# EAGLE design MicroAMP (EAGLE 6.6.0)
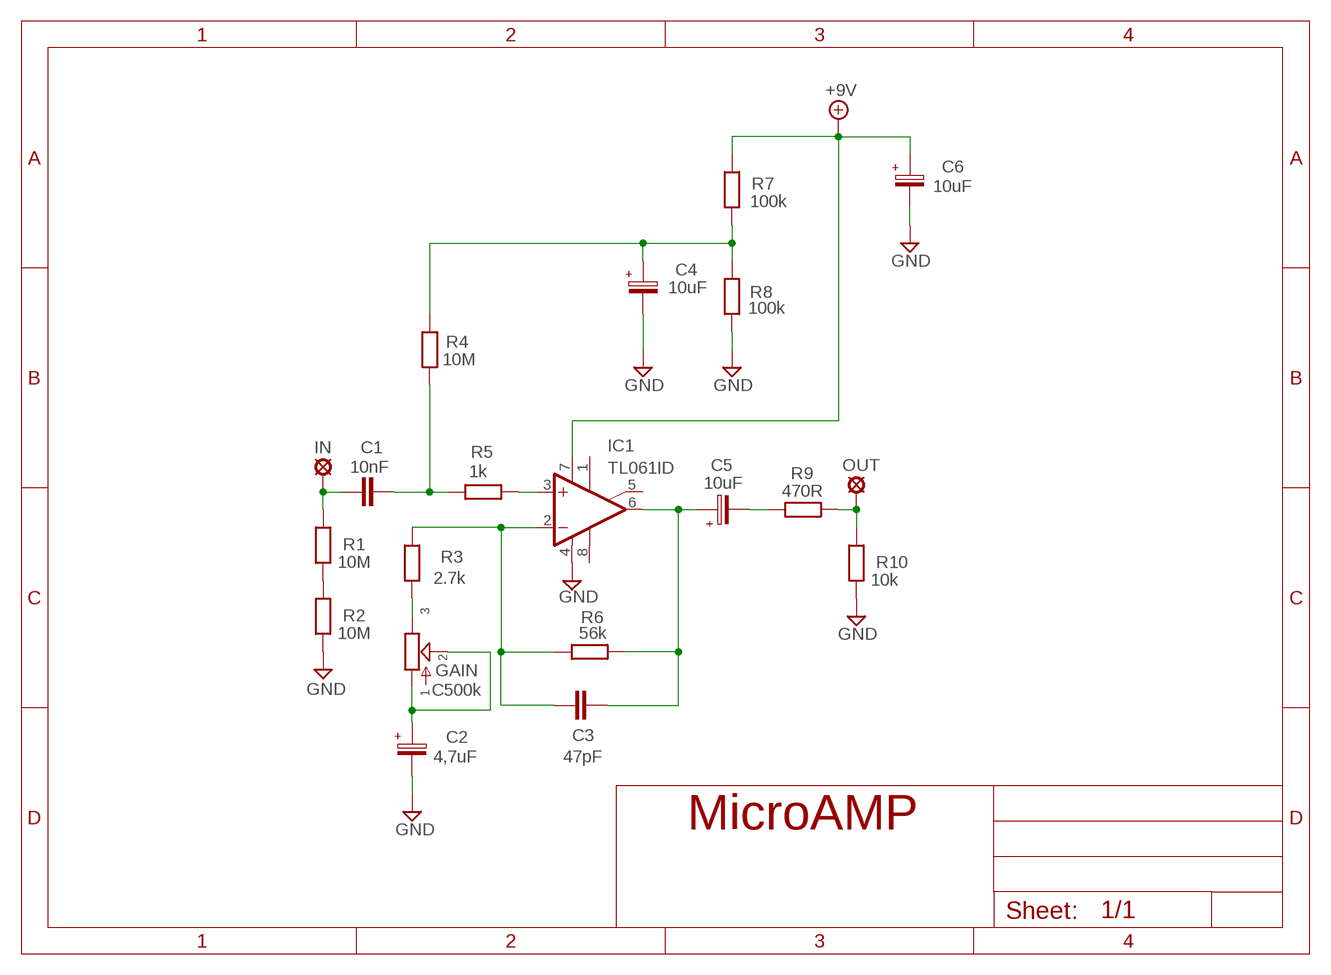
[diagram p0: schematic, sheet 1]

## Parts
+9V  +9V  +9V(T)1  [ROUND]
C1  10nF  1NF-15NF  [3,5MM]
C2  4,7uF  063-EU  [063_025]
C3  47pF  050X030_0501  [050X030_050_1]
C4  10uF  063-EU  [063_025]
C5  10uF  063-EU  [063_025]
C6  10uF  063-EU  [063_025]
GAIN  C500k  POT-EU16MM  [16MM]
GND  GND  GND(T)1  [ROUND]
GND7  GND  GND(T)1  [ROUND]
IC1  TL061ID  TL071D  [SO08]
IN  MCS10B  [MCS10B]
OUT  MCS10B  [MCS10B]
R1  10M  6MM-EU3  [R0207/3]
R2  10M  6MM-EU3  [R0207/3]
R3  2.7k  6MM-EU3  [R0207/3]
R4  10M  6MM-EU3  [R0207/3]
R5  1k  6MM-EU3  [R0207/3]
R6  56k  6MM-EU3  [R0207/3]
R7  100k  6MM-EU3  [R0207/3]
R8  100k  6MM-EU3  [R0207/3]
R9  470R  6MM-EU3  [R0207/3]
R10  10k  6MM-EU3  [R0207/3]

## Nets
+9V: +9V.1(+9V) C6.+ IC1.7(V+) R7.2
GND: C2.- C4.- C6.- GND7.1(GND) GND.1(GND) IC1.4(V-) R2.1 R8.1 R10.1
N$1: GAIN.3 R3.1
N$2: C5.- R9.1
N$3: C4.+ R4.2 R7.1 R8.2
N$5: C1.2 R4.1 R5.1
N$6: IC1.3(+IN) R5.2
N$7: C3.2 C5.+ IC1.6(OUT) R6.2
N$8: C2.+ GAIN.1 GAIN.2
N$9: C3.1 IC1.2(-IN) R3.2 R6.1
N$11: C1.1 IN.MP R1.2
N$12: R1.1 R2.2
N$13: OUT.MP R9.2 R10.2
Unconnected: IC1.1(ON1) IC1.5(ON2) IC1.8(OPT)

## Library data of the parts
+9V = gm-supply:+9V(T): +9V Voltage Supply
C1 = Mylar Kondensaattorit:1NF-15NF: 1nF-15nF
C2 C4-C6 = Elektrolyytit:063-EU
C3 = Keraamiset kondensaattorit:050X030_050: 120 - 150pF
GAIN = gm-pots:POT-EU
GND GND7 = gm-supply:GND(T): Ground
IC1 = gm-ics:TL071: OP AMP
IN OUT = Padit:MCS10B: SOLDER PAD
R1-R10 = Vastukset:6MM-EU: 6mm Resistors (European schematic symbol)

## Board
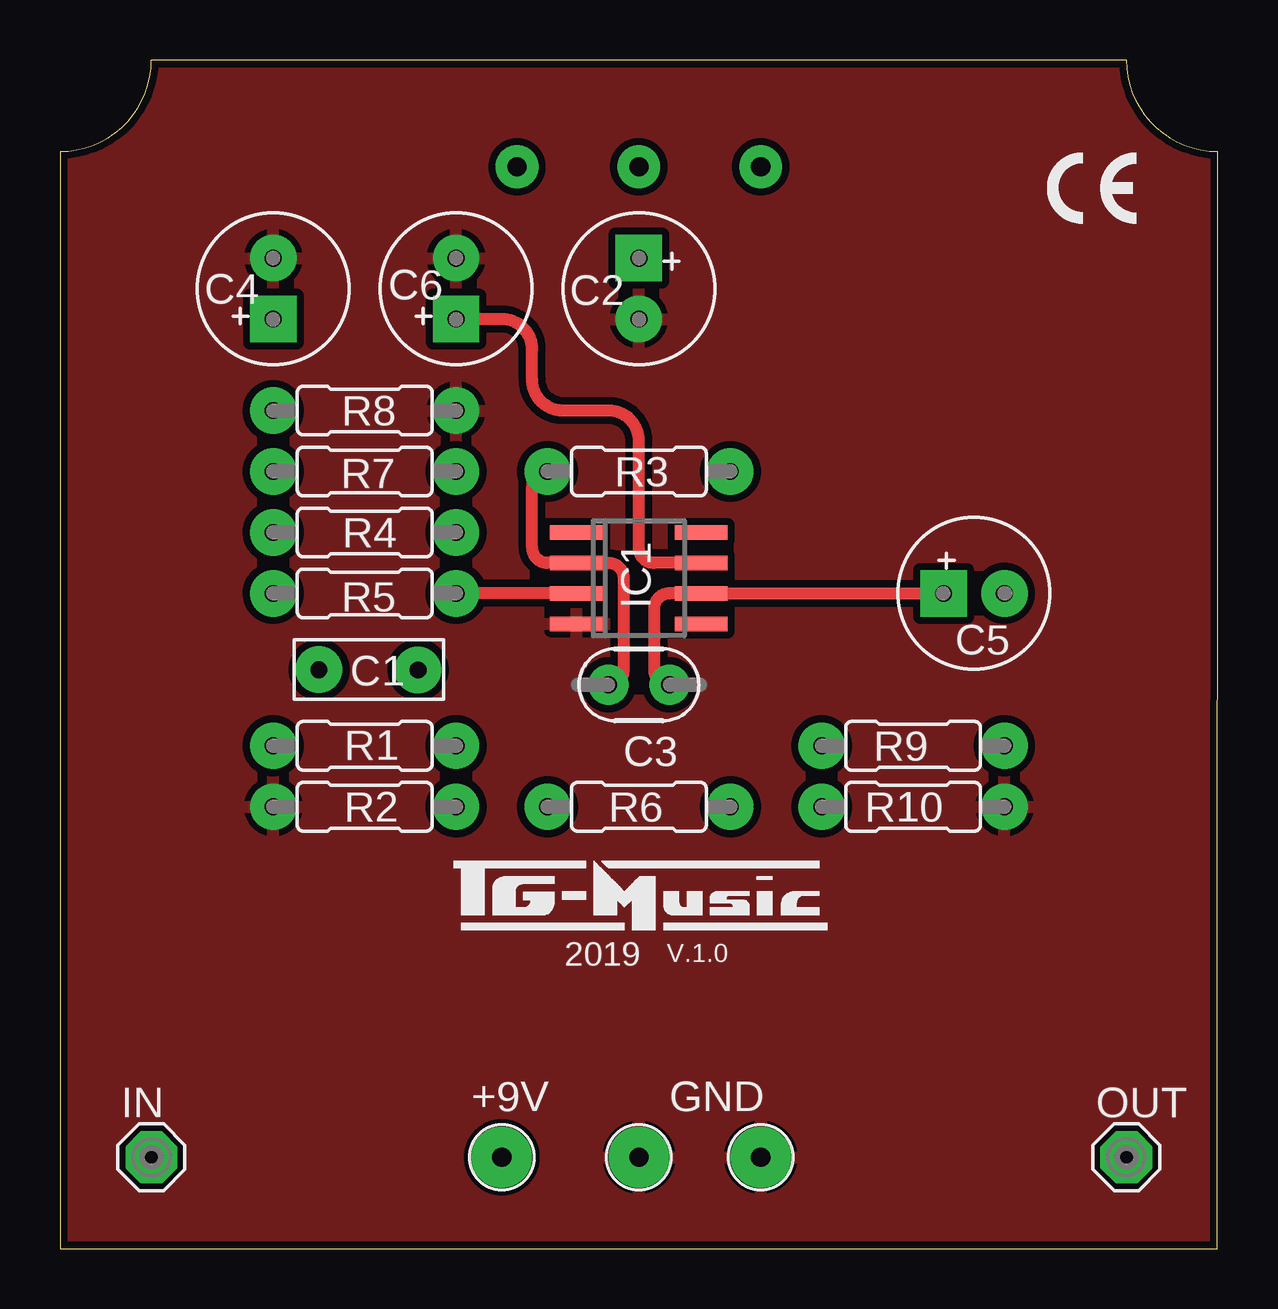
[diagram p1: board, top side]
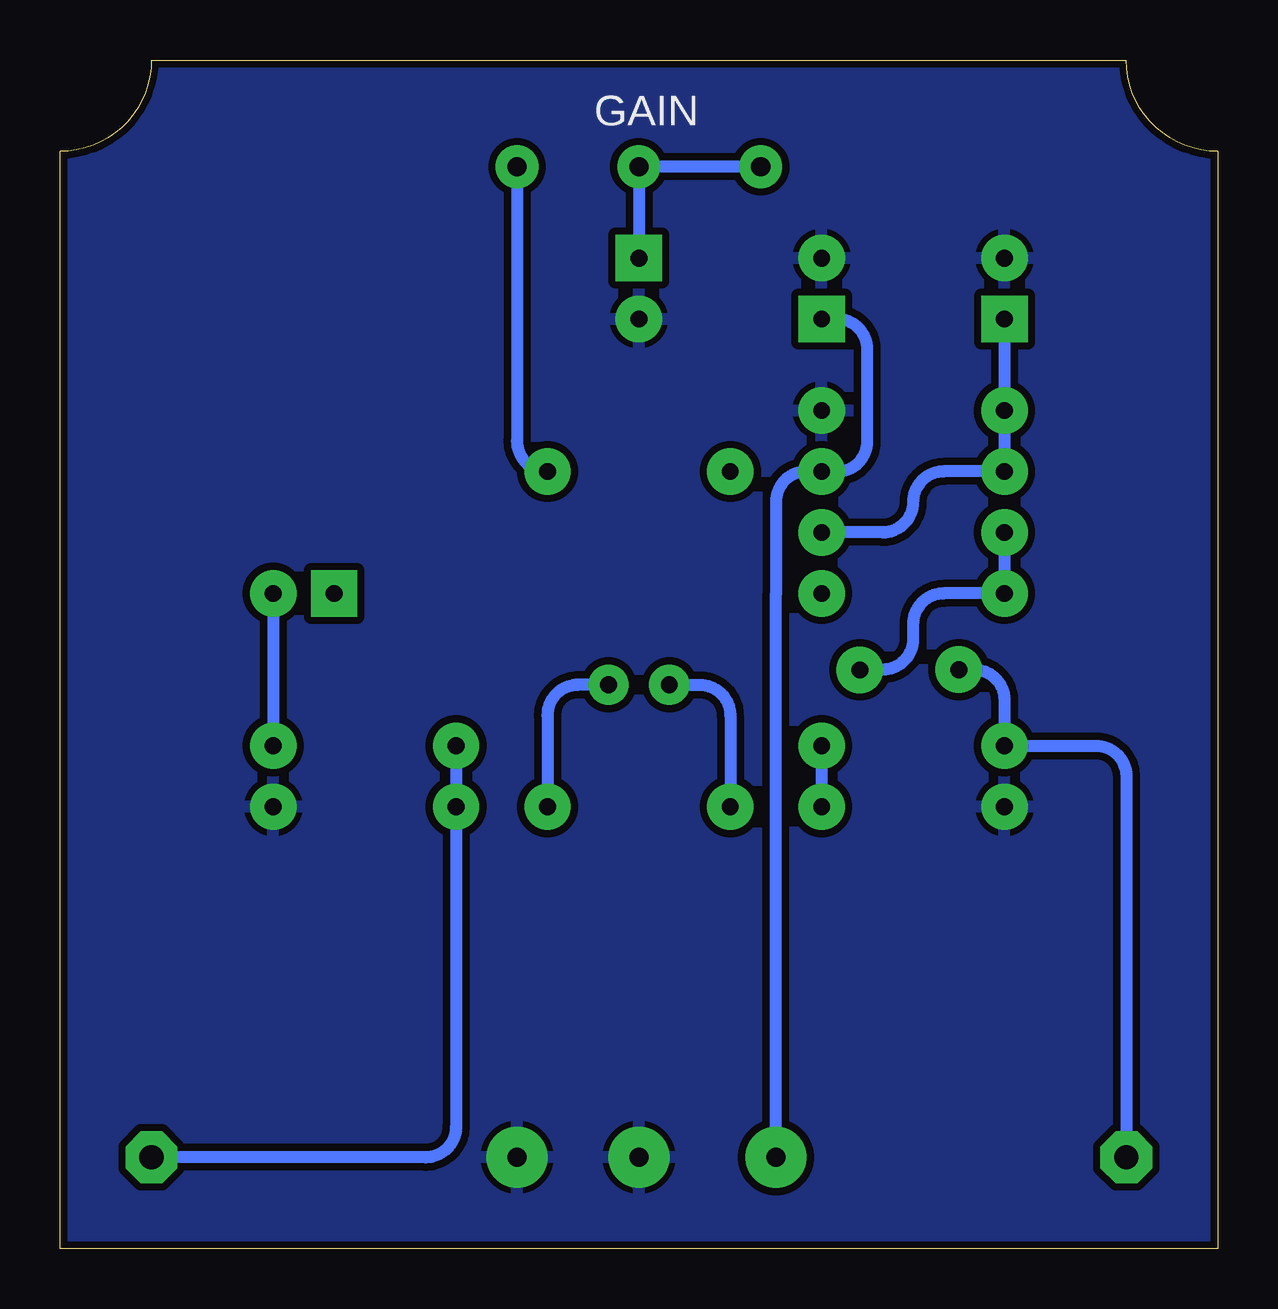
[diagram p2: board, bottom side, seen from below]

Size 48.26 x 49.53 mm. Coordinates in mm from the lower left corner, seen from the top.
Outline: 48.26,45.72 48.24,0 0,0 0,45.72
Outline: 3.81,49.53 7.62,49.53 44.45,49.53 arc90 48.26,45.72
Outline: 0,45.72 arc90 3.81,49.53
Copper layers (1*16): Top 0.035mm / dielectric 1.5mm / Bottom 0.035mm
Design rules "ITEADstudio": minimum track width 10mil, minimum drill 12mil, track to track 12mil, track to pad 12mil, pad to pad 12mil, via to via 12mil, smd to smd 0mil, copper to edge 12mil, drill to drill 12mil, minimum pad ring 10mil, minimum via ring 6mil, stop-mask expansion 4mil, vias tented up to drill 100mil, thermal gap 10mil

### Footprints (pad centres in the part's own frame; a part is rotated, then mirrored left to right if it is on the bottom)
ROUND = drill 0.8 pad 2.54: 1 0,0
3,5MM = drill 0.7 pad 1.93: 1 -1.905,0; 2 2.221,-0.016
063_025 = drill 0.7 pad 1.93 square: + -1.27,0 | drill 0.7 pad 1.93: - 1.27,0
050X030_050_1 = drill 0.7 pad 1.676: 1 -1.27,0; 2 1.27,0
16MM = drill 0.8 pad 1.778: 1 5.08,0; 2 0,0; 3 -5.08,0
SO08 = smd 0.6 x 2.2: 1 -1.905,-2.6; 2 -0.635,-2.6; 3 0.635,-2.6; 4 1.905,-2.6; 5 1.905,2.6; 6 0.635,2.6; 7 -0.635,2.6; 8 -1.905,2.6
MCS10B = drill 1.016 pad 2.159 octagon: MP 0,0
R0207/3 = drill 0.7 pad 1.93: 1 -3.81,0; 2 3.81,0

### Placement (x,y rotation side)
+9V  18.42,3.81 0 top
C1  12.7,24.13 0 top
C2  24.13,40.01 270 top
C3  24.13,23.5 0 top
C4  8.89,40.01 90 top
C5  38.1,27.3 0 top
C6  16.51,40.01 90 top
GAIN  24.13,45.09 0 bottom
GND  24.13,3.81 0 top
GND7  29.21,3.81 0 top
IC1  24.13,27.94 270 top
IN  3.81,3.81 0 top
OUT  44.45,3.81 0 top
R1  12.7,20.95 180 top
R2  12.7,18.41 0 top
R3  24.13,32.38 180 top
R4  12.7,29.84 0 top
R5  12.7,27.3 0 top
R6  24.13,18.41 0 top
R7  12.7,32.38 0 top
R8  12.7,34.92 180 top
R9  35.56,20.95 180 top
R10  35.56,18.41 180 top

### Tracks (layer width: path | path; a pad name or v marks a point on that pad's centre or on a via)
+9V
  Top 0.508: IC1.7 24.77,28.57 arc-90 24.13,29.21 24.13,33.66 arc90 22.86,34.92 20.96,34.92 arc-90 19.69,36.2 19.69,37.47 arc90 18.42,38.73 C6.+
  Bottom 0.508: C6.+ 15.88,38.73 arc90 14.61,37.47 14.61,33.66 arc90 15.88,32.38 R7.2 17.15,32.38 arc-90 18.42,31.11 18.42,27.3 +9V.1
GND
  pour Top: 0,0 0,45.72 arc-90 3.81,49.53 44.45,49.53 arc-90 48.26,45.72 48.26,0
  pour Bottom: 0,0 0,45.72 arc-90 3.81,49.53 44.45,49.53 arc-90 48.26,45.72 48.26,0
N$1
  Bottom 0.508: GAIN.3 29.21,33.66 arc-90 R3.1
N$2
  Bottom 0.508: C5.- R9.1
N$3
  Bottom 0.508: C4.+ R8.2 R7.1 11.43,32.38 arc-90 12.7,31.11 arc90 13.97,29.84 R4.2
N$5
  Bottom 0.508: R4.1 R5.1 11.43,27.3 arc-90 12.7,26.04 12.7,25.4 arc90 13.97,24.13 14.91,24.13 arc-90 C1.2
N$6
  Top 0.508: IC1.3 R5.2
N$7
  Top 0.508: C5.+ 31.12,27.3 IC1.6 25.4,27.3 arc90 24.77,26.67 24.77,24.13 arc90 C3.2
  Bottom 0.508: C3.2 26.67,23.5 arc-90 27.94,22.23 R6.2
N$8
  Bottom 0.508: GAIN.1 GAIN.2 C2.+
N$9
  Top 0.508: R3.2 arc90 19.69,31.75 19.69,29.21 arc90 20.32,28.57 IC1.2 22.86,28.57 arc-90 23.5,27.94 23.5,24.13 arc-90 C3.1
  Bottom 0.508: C3.1 21.59,23.5 arc90 20.32,22.23 R6.1
N$11
  Bottom 0.508: C1.1 10.16,24.13 arc90 8.89,22.86 R1.2 5.08,20.95 arc90 3.81,19.68 IN.MP
N$12
  Bottom 0.508: R1.1 R2.2
N$13
  Bottom 0.508: R9.2 R10.2 31.75,5.08 arc90 33.02,3.81 OUT.MP

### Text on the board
tNames: 2019 | V.1.0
